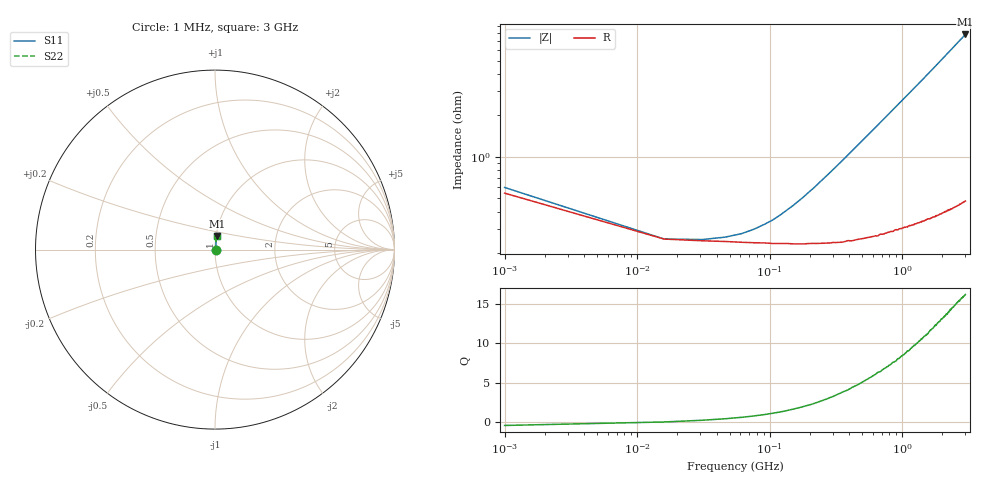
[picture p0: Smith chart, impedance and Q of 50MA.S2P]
!Keysight Technologies,E4991B,MY54301043,A.02.04
!Date: Thu Nov 16 21:15:29 2023
!Data:
!Freq	S11	S21	S12	S22
# Hz S MA R 50
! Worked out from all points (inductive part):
!   201 points, 1 MHz to 3 GHz, reference 50 ohm
!   read as one part in series: L = 410 pH near 285.9 MHz
!   highest Q = 16.2 at 3 GHz (marker M1), where L = 411 pH
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1000000  0.005962 -24.5  0.9946 0.1  0.9946 0.1  0.005962 -24.5
1.5995e7  0.002521 -0.7  0.9975 0.0  0.9975 0.0  0.002521 -0.7
3.099e7  0.002501 11.6  0.9976 -0.0  0.9976 -0.0  0.002501 11.6
4.5985e7  0.002602 21.5  0.9976 -0.1  0.9976 -0.1  0.002602 21.5
6.098e7  0.002756 29.8  0.9976 -0.1  0.9976 -0.1  0.002756 29.8
1.35955e8  0.004119 55.2  0.9977 -0.2  0.9977 -0.2  0.004119 55.2
1.65945e8  0.004781 60.6  0.9977 -0.2  0.9977 -0.2  0.004781 60.6
1.95935e8  0.005489 64.5  0.9976 -0.3  0.9976 -0.3  0.005489 64.5
2.55915e8  0.006941 69.8  0.9976 -0.4  0.9976 -0.4  0.006941 69.8
3.15895e8  0.008441 73.2  0.9976 -0.5  0.9976 -0.5  0.008441 73.2
3.9087e8  0.01034 75.7  0.9975 -0.6  0.9975 -0.6  0.01034 75.7
5.1083e8  0.01337 78.3  0.9974 -0.8  0.9974 -0.8  0.01337 78.3
6.15795e8  0.016 79.6  0.9972 -0.9  0.9972 -0.9  0.016 79.6
7.35755e8  0.01901 80.6  0.9971 -1.1  0.9971 -1.1  0.01901 80.6
8.85705e8  0.02279 81.3  0.9968 -1.3  0.9968 -1.3  0.02279 81.3
1.005665e9  0.02579 81.8  0.9966 -1.5  0.9966 -1.5  0.02579 81.8
1.245585e9  0.03183 82.3  0.9962 -1.8  0.9962 -1.8  0.03183 82.3
1.5005e9  0.03826 82.6  0.9958 -2.2  0.9958 -2.2  0.03826 82.6
1.74042e9  0.04437 82.7  0.9954 -2.5  0.9954 -2.5  0.04437 82.7
2.01033e9  0.05128 82.7  0.9948 -2.9  0.9948 -2.9  0.05128 82.7
2.505165e9  0.06409 82.5  0.9936 -3.7  0.9936 -3.7  0.06409 82.5
3e9  0.07697 82.1  0.9923 -4.4  0.9923 -4.4  0.07697 82.1
